|   TEXAS INSTRUMENTS INCORPORATED
|   Standard Linear and Logic
|   IBIS Model of SN74LVTH16501
|   18 Bit Universal Bus Transceiver
|   TSSOP 56 pin package(DGG)
|   SSOP 56 pin package(DL)
[IBIS Ver]   2.1
[Comment char]   |_char
[File Name]   sn74lvth16501.ibs
[File Rev]   1.0
[Date]   07-17-2000
[Source]   File originated at Texas Instruments, Inc
[Notes]   The following is an IBIS list for LVTH16501.
   - All test data contained in this file are derived from hspice
   (tm) simulations.
   - This file may be incomplete or may not be fully compliant
   with the IBIS specification. It will be replaced with a
   version that is IBIS Revision 3.2 compliant and is complete
   and accurate. Please email all questions and comments to
   sllibis@ti.com.
|   -For Questions or Comments please mailto:sllibis@ti.com
|*   Property of Texas Instruments Incorporated.  Unauthorized   *
|*   reproduction and/or distribution is strictly prohibited.   *
|*   This product is protected under copyright law.   *
|*   Created 1998, (C) Copyright 1998, Texas Instruments Inc.,   *
|*   All Rights Reserved   *
|*   UNLESS THERE IS A SIGNED, WRITTEN AGREEMENT TO THE   *
|*   CONTRARY, TEXAS INSTRUMENTS ("TI") IS PROVIDING THE SPICE   *
|*   MODELS "AS IS" AND WITHOUT ANY WARRANTY, EXPRESSED OR   *
|*   IMPLIED.  TI assumes no liability for:   *
|*   1) the accuracy of the IBIS models provided to your   *
|*   company;   *
|*   2) the proper functioning of these IBIS models in your   *
|*   design or for any resulting applications; or   *
|*   3) infringement of patents, copyrights or intellectual   *
|*   property rights resulting from your use of these   *
|*   IBIS models.   *
|*   TI provides IBIS Models as a service to our customers.   *
|*   You and your company shall not distribute, sell or give   *
|*   these models to anyone else without prior written   *
|*   permission from TI.   *
|*   TI reserves the right to make changes to our products or   *
|*   to discontinue any semiconductor product or service   *
|*   without notice, and advises our customers to obtain the   *
|*   latest version of relevant information to verify, before   *
|*   placing orders, that the information being relied on is   *
|*   current.   *
|*   Please be aware that your receipt and use of the IBIS   *
|*   information provided shall serve as acceptance of these   *
|*   terms and conditions.  If you do not accept these terms,   *
|*   you should return or destroy the IBIS models and any   *
|*   other accompanying information immediately.   *
|   TSSOP PACKAGE (DGG)
[Component]   LVTH16501_DGG
[manufacturer]   Texas Instruments, Inc.
[Package]
|   typ   min   max
R_pkg   0.045   0.035   0.062
L_pkg   3.324nH   2.403nH   5.094nH
C_pkg   0.564pF   0.341pF   0.914nH
[Pin]   signal_name   model_name   R_pin   L_pin   C_pin
1   OEAB   LVTH16501_OEAB   0.062   5.094nH   0.856pF
2   LEAB   LVTH16501_IN   0.061   4.621nH   0.902pF
3   A1   LVTH16501_I_O   0.06   4.316nH   0.802pF
4   GND   GND   0.059   3.968nH   0.698pF
5   A2   LVTH16501_I_O   0.057   3.716nH   0.649pF
6   A3   LVTH16501_I_O   0.042   3.517nH   0.652pF
7   VCC   POWER   0.041   3.16nH   0.57pF
8   A4   LVTH16501_I_O   0.039   2.981nH   0.482pF
9   A5   LVTH16501_I_O   0.039   2.809nH   0.447pF
10   A6   LVTH16501_I_O   0.038   2.715nH   0.409pF
11   GND   GND   0.041   2.675nH   0.391pF
12   A7   LVTH16501_I_O   0.039   2.536nH   0.366pF
13   A8   LVTH16501_I_O   0.039   2.457nH   0.348pF
14   A9   LVTH16501_I_O   0.038   2.411nH   0.353pF
15   A10   LVTH16501_I_O   0.039   2.456nH   0.355pF
16   A11   LVTH16501_I_O   0.039   2.471nH   0.349pF
17   A12   LVTH16501_I_O   0.04   2.58nH   0.37pF
18   GND   GND   0.038   2.651nH   0.389pF
19   A13   LVTH16501_I_O   0.038   2.739nH   0.411pF
20   A14   LVTH16501_I_O   0.039   2.838nH   0.449pF
21   A15   LVTH16501_I_O   0.038   2.988nH   0.484pF
22   VCC   POWER   0.038   3.105nH   0.564pF
23   A16   LVTH16501_I_O   0.04   3.427nH   0.638pF
24   A17   LVTH16501_I_O   0.056   3.654nH   0.641pF
25   GND   GND   0.057   3.932nH   0.7pF
26   A18   LVTH16501_I_O   0.058   4.257nH   0.806pF
27   NOEBA   LVTH16501_NOEBA   0.057   4.58nH   0.914pF
28   LEBA   LVTH16501_IN   0.059   5.038nH   0.861pF
29   GND   GND   0.06   5.058nH   0.858pF
30   CLKBA   LVTH16501_IN   0.056   4.543nH   0.904pF
31   B18   LVTH16501_I_O   0.057   4.24nH   0.803pF
32   GND   GND   0.057   3.929nH   0.7pF
33   B17   LVTH16501_I_O   0.056   3.616nH   0.637pF
34   B16   LVTH16501_I_O   0.037   3.368nH   0.64pF
35   VCC   POWER   0.036   3.024nH   0.563pF
36   B15   LVTH16501_I_O   0.035   2.876nH   0.474pF
37   B14   LVTH16501_I_O   0.035   2.745nH   0.444pF
38   B13   LVTH16501_I_O   0.037   2.683nH   0.405pF
39   GND   GND   0.038   2.603nH   0.382pF
40   B12   LVTH16501_I_O   0.038   2.51nH   0.362pF
41   B11   LVTH16501_I_O   0.036   2.412nH   0.341pF
42   B10   LVTH16501_I_O   0.038   2.416nH   0.349pF
43   B9   LVTH16501_I_O   0.037   2.403nH   0.349pF
44   B8   LVTH16501_I_O   0.037   2.429nH   0.341pF
45   B7   LVTH16501_I_O   0.036   2.482nH   0.358pF
46   GND   GND   0.037   2.615nH   0.381pF
47   B6   LVTH16501_I_O   0.035   2.669nH   0.402pF
48   B5   LVTH16501_I_O   0.036   2.763nH   0.442pF
49   B4   LVTH16501_I_O   0.036   2.942nH   0.478pF
50   VCC   POWER   0.035   3.053nH   0.564pF
51   B3   LVTH16501_I_O   0.036   3.409nH   0.641pF
52   B2   LVTH16501_I_O   0.058   3.698nH   0.641pF
53   GND   GND   0.059   3.975nH   0.697pF
54   B1   LVTH16501_I_O   0.061   4.327nH   0.802pF
55   CLKAB   LVTH16501_IN   0.061   4.624nH   0.905pF
56   GND   GND   0.06   5.063nH   0.858pF
|   SSOP PACKAGE (DL)
[Component]   LVTH16501_DL
[manufacturer]   Texas Instruments, Inc.
[Package]
|   typ   min   max
R_pkg   0.055   0.048   0.067
L_pkg   6.539nH   4.802nH   9.746nH
C_pkg   0.85pF   0.5pF   1.351pF
[Pin]   signal_name   model_name   R_pin   L_pin   C_pin
1   OEAB   LVTH16501_OEAB   0.064   9.646nH   1.202pF
2   LEAB   LVTH16501_IN   0.059   8.723nH   1.348pF
3   A1   LVTH16501_I_O   0.059   8.139nH   1.223pF
4   GND   GND   0.056   7.554nH   1.088pF
5   A2   LVTH16501_I_O   0.054   6.991nH   0.966pF
6   A3   LVTH16501_I_O   0.053   6.659nH   0.973pF
7   VCC   POWER   0.055   6.321nH   0.905pF
8   A4   LVTH16501_I_O   0.055   5.942nH   0.713pF
9   A5   LVTH16501_I_O   0.057   5.767nH   0.678pF
10   A6   LVTH16501_I_O   0.054   5.459nH   0.631pF
11   GND   GND   0.051   5.224nH   0.638pF
12   A7   LVTH16501_I_O   0.048   5.088nH   0.601pF
13   A8   LVTH16501_I_O   0.05   5.021nH   0.518pF
14   A9   LVTH16501_I_O   0.051   4.802nH   0.5pF
15   A10   LVTH16501_I_O   0.051   4.803nH   0.5pF
16   A11   LVTH16501_I_O   0.05   5.021nH   0.518pF
17   A12   LVTH16501_I_O   0.048   5.088nH   0.601pF
18   GND   GND   0.051   5.224nH   0.638pF
19   A13   LVTH16501_I_O   0.054   5.459nH   0.631pF
20   A14   LVTH16501_I_O   0.057   5.768nH   0.677pF
21   A15   LVTH16501_I_O   0.055   5.942nH   0.715pF
22   VCC   POWER   0.055   6.321nH   0.907pF
23   A16   LVTH16501_I_O   0.053   6.659nH   0.972pF
24   A17   LVTH16501_I_O   0.054   6.991nH   0.966pF
25   GND   GND   0.056   7.554nH   1.087pF
26   A18   LVTH16501_I_O   0.059   8.139nH   1.223pF
27   NOEBA   LVTH16501_NOEBA   0.059   8.727nH   1.351pF
28   LEBA   LVTH16501_IN   0.067   9.746nH   1.21pF
29   GND   GND   0.063   9.63nH   1.203pF
30   CLKBA   LVTH16501_IN   0.06   8.751nH   1.349pF
31   B18   LVTH16501_I_O   0.06   8.184nH   1.224pF
32   GND   GND   0.056   7.543nH   1.087pF
33   B17   LVTH16501_I_O   0.054   7.005nH   0.969pF
34   B16   LVTH16501_I_O   0.056   6.714nH   0.975pF
35   VCC   POWER   0.058   6.384nH   0.909pF
36   B15   LVTH16501_I_O   0.057   5.976nH   0.717pF
37   B14   LVTH16501_I_O   0.057   5.743nH   0.677pF
38   B13   LVTH16501_I_O   0.055   5.469nH   0.631pF
39   GND   GND   0.055   5.328nH   0.644pF
40   B12   LVTH16501_I_O   0.052   5.189nH   0.606pF
41   B11   LVTH16501_I_O   0.052   5.053nH   0.519pF
42   B10   LVTH16501_I_O   0.052   4.825nH   0.502pF
43   B9   LVTH16501_I_O   0.054   4.896nH   0.506pF
44   B8   LVTH16501_I_O   0.052   5.093nH   0.521pF
45   B7   LVTH16501_I_O   0.051   5.179nH   0.608pF
46   GND   GND   0.054   5.314nH   0.645pF
47   B6   LVTH16501_I_O   0.055   5.511nH   0.632pF
48   B5   LVTH16501_I_O   0.057   5.77nH   0.677pF
49   B4   LVTH16501_I_O   0.055   5.956nH   0.716pF
50   VCC   POWER   0.055   6.32nH   0.905pF
51   B3   LVTH16501_I_O   0.052   6.621nH   0.968pF
52   B2   LVTH16501_I_O   0.053   6.974nH   0.966pF
53   GND   GND   0.057   7.571nH   1.089pF
54   B1   LVTH16501_I_O   0.057   8.097nH   1.219pF
55   CLKAB   LVTH16501_IN   0.059   8.723nH   1.349pF
56   GND   GND   0.061   9.56nH   1.199pF
| Models and submodels in the file (4): LVTH16501_I_O (I/O), LVTH16501_OEAB (Input), LVTH16501_NOEBA (Input), LVTH16501_IN (Input)
